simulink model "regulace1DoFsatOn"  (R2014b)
settings: Solver=ode45  StartTime=0.0  StopTime=50  RelTol=1e-3
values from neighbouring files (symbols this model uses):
  p = [0.2728 0.1079 0.3077 0.0546]    [SITOrizeniP.m]    (also in SITOrizeniPD.m; normaHnekonecno.m = [1 (3*alfa(j)-a0)])
  par = [0.2728 0.1079 0.3077 0.0546 0.1370 0.0320 0.1151 0.0357]    [regulace1DoF.m]    (also in SITOrizeniP.m = [-0.0536 0.05 0.13 0.006 -0.0545 0.1 0.16 0.1746 -0.058     ; SITOrizeniPD.m = [-0.0536 0.05 0.13 0.006 -0.0545 0.1 0.16 0.1746 -0.058     ; regulace2DoF.m; regulaceMPM.m)
undefined symbols (not defined in the file or in its folder): magnitude, q
libraries: simulink x4

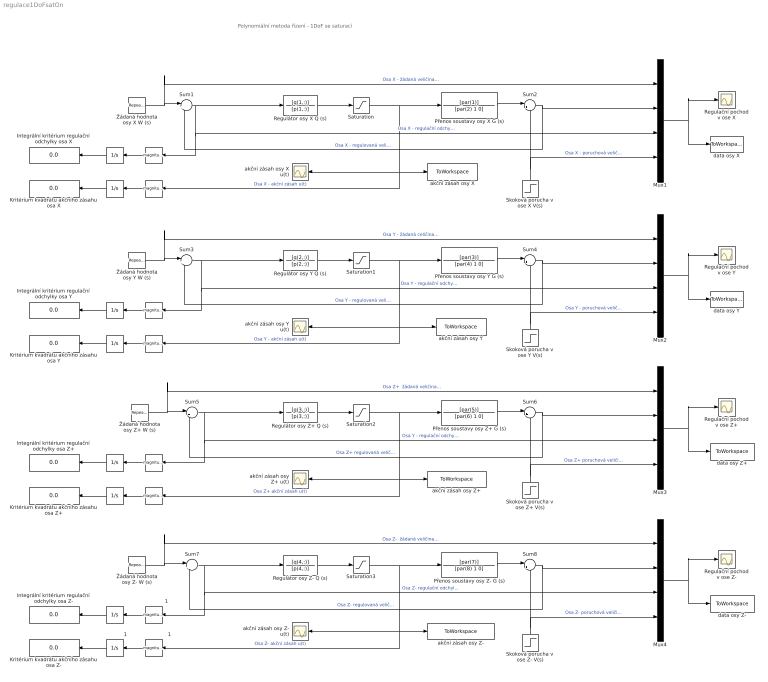
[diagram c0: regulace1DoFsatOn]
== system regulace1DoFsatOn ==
  note: Polynomiální metoda řízení - 1DoF se saturací
  " " : Math  Operator=magnitude^2
  "  " : Integrator
  "    " : Integrator
  "     " : Integrator
  "      " : Math  Operator=magnitude^2
  "        " : Integrator
  "         " : Integrator
  "          " : Math  Operator=magnitude^2
  "             " : Math  Operator=magnitude^2
  "              " : Integrator
  "                 " : Math  Operator=magnitude^2
  "                     " : Math  Operator=magnitude^2
  "                                                  " : Integrator
  "                     1" : Math  Operator=magnitude^2
  "                 1" : Math  Operator=magnitude^2
  "              1" : Integrator
  Integrální kritérium regulační odchylky osa X : Display
  Integrální kritérium regulační odchylky osa Y : Display
  Integrální kritérium regulační odchylky osa Z+ : Display
  Integrální kritérium regulační odchylky osa Z- : Display
  Kritérium kvadrátu akčního zásahu osa X : Display
  Kritérium kvadrátu akčního zásahu osa Y : Display
  Kritérium kvadrátu akčního zásahu osa Z+ : Display
  Kritérium kvadrátu akčního zásahu osa Z- : Display
  Mux{1..4} (4 alike) : Mux
  Přenos soustavy osy X G (s) : TransferFcn  Numerator=[par(1)]  Denominator=[par(2) 1 0]
  Přenos soustavy osy Y G (s) : TransferFcn  Numerator=[par(3)]  Denominator=[par(4) 1 0]
  Přenos soustavy osy Z+ G (s) : TransferFcn  Numerator=[par(5)]  Denominator=[par(6) 1 0]
  Přenos soustavy osy Z- G (s) : TransferFcn  Numerator=[par(7)]  Denominator=[par(8) 1 0]
  Regulační pochod v ose X : Scope
  Regulační pochod v ose Y : Scope
  Regulační pochod v ose Z+ : Scope
  Regulační pochod v ose Z- : Scope
  Regulátor osy X Q (s) : TransferFcn  Numerator=[q(1,:)]  Denominator=[p(1,:)]
  Regulátor osy Y Q (s) : TransferFcn  Numerator=[q(2,:)]  Denominator=[p(2,:)]
  Regulátor osy Z+ Q (s) : TransferFcn  Numerator=[q(3,:)]  Denominator=[p(3,:)]
  Regulátor osy Z- Q (s) : TransferFcn  Numerator=[q(4,:)]  Denominator=[p(4,:)]
  Saturation{,1..3} (4 alike) : Saturate  UpperLimit=1  LowerLimit=-1
  Skoková porucha v ose X V(s) : Step  Time=15  After=0.1  SampleTime=0
  Skoková porucha v ose Y V(s) : Step  Time=15  After=0.1  SampleTime=0
  Skoková porucha v ose Z+ V(s) : Step  Time=15  After=0.1  SampleTime=0
  Skoková porucha v ose Z- V(s) : Step  Time=15  After=0.1  SampleTime=0
  Sum{1,3,5,7} (4 alike) : Sum  Inputs=|+-
  Sum{2,4,6,8} (4 alike) : Sum  Inputs=|++
  akční zásah osy X : ToWorkspace  VariableName=akcniZasahXsat  SaveFormat=Timeseries  SampleTime=-1
  akční zásah osy X u(t) : Scope
  akční zásah osy Y : ToWorkspace  VariableName=akcniZasahYsat  SaveFormat=Timeseries  SampleTime=-1
  akční zásah osy Y u(t) : Scope
  akční zásah osy Z+ : ToWorkspace  VariableName=akcniZasahZplusSat  SaveFormat=Timeseries  SampleTime=-1
  akční zásah osy Z+ u(t) : Scope
  akční zásah osy Z- : ToWorkspace  VariableName=akcniZasahZminusSat  SaveFormat=Timeseries  SampleTime=-1
  akční zásah osy Z- u(t) : Scope
  data osy X : ToWorkspace  VariableName=dataXsat  SaveFormat=Timeseries  SampleTime=-1
  data osy Y : ToWorkspace  VariableName=dataYsat  SaveFormat=Timeseries  SampleTime=-1
  data osy Z+ : ToWorkspace  VariableName=dataZplusSat  SaveFormat=Timeseries  SampleTime=-1
  data osy Z- : ToWorkspace  VariableName=dataZminusSat  SaveFormat=Timeseries  SampleTime=-1
  Žádaná hodnota osy X W (s) : simulink/Sources/Repeating Sequence  rep_seq_t=[0 9.99 10 19.99 20 29.99 30 39.99 40 50]  rep_seq_y=[0 0 0.4 0.4 0.2 0.2 0.6 0.6 0 0]
  Žádaná hodnota osy Y W (s) : simulink/Sources/Repeating Sequence  rep_seq_t=[0 9.99 10 19.99 20 29.99 30 39.99 40 50]  rep_seq_y=[0 0 0.4 0.4 0.2 0.2 0.6 0.6 0 0]
  Žádaná hodnota osy Z+ W (s) : simulink/Sources/Repeating Sequence  rep_seq_t=[0 9.99 10 19.99 20 29.99 30 39.99 40 50]  rep_seq_y=[0 0 0.4 0.4 0.2 0.2 0.6 0.6 0 0]
  Žádaná hodnota osy Z- W (s) : simulink/Sources/Repeating Sequence  rep_seq_t=[0 9.99 10 19.99 20 29.99 30 39.99 40 50]  rep_seq_y=[0 0 0.4 0.4 0.2 0.2 0.6 0.6 0 0]
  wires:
  Žádaná hodnota osy X W (s)/1 -> Sum1/1, Mux1/1  "Osa X - žádaná veličina w(t)"
  Sum1/1 -> Regulátor osy X Q (s)/1, Mux1/3, "      "/1  "Osa X - regulační odchylka e(t)"
  Přenos soustavy osy X G (s)/1 -> Sum2/1
  Sum2/1 -> Sum1/2, Mux1/2  "Osa X - regulovaná veličina y(t)"
  Skoková porucha v ose X V(s)/1 -> Mux1/4, Sum2/2  "Osa X - poruchová veličina v(t)"
  Mux1/1 -> data osy X/1, Regulační pochod v ose X/1
  "      "/1 -> "  "/1
  "  "/1 -> Integrální kritérium regulační odchylky osa X/1
  "     "/1 -> Kritérium kvadrátu akčního zásahu osa X/1
  " "/1 -> "     "/1
  Saturation/1 -> Přenos soustavy osy X G (s)/1, akční zásah osy X/1, " "/1, akční zásah osy X u(t)/1  "Osa X - akční zásah u(t)"
  Regulátor osy X Q (s)/1 -> Saturation/1
  Žádaná hodnota osy Y W (s)/1 -> Sum3/1, Mux2/1  "Osa Y - žádaná celičina w(t)"
  Sum3/1 -> Regulátor osy Y Q (s)/1, Mux2/3, "          "/1  "Osa Y - regulační odchylka e(t)"
  Přenos soustavy osy Y G (s)/1 -> Sum4/1
  Sum4/1 -> Sum3/2, Mux2/2  "Osa Y - regulovaná veličina y(t)"
  Skoková porucha v ose Y V(s)/1 -> Mux2/4, Sum4/2  "Osa Y - poruchová veličina v(t)"
  Mux2/1 -> data osy Y/1, Regulační pochod v ose Y/1
  "          "/1 -> "    "/1
  "    "/1 -> Integrální kritérium regulační odchylky osa Y/1
  "        "/1 -> Kritérium kvadrátu akčního zásahu osa Y/1
  "             "/1 -> "        "/1
  Saturation1/1 -> Přenos soustavy osy Y G (s)/1, akční zásah osy Y/1, "             "/1, akční zásah osy Y u(t)/1  "Osa Y - akční zásah u(t)"
  Regulátor osy Y Q (s)/1 -> Saturation1/1
  Žádaná hodnota osy Z+ W (s)/1 -> Sum5/1, Mux3/1  "Osa Z+  žádaná veličina w(t)"
  Sum5/1 -> Regulátor osy Z+ Q (s)/1, Mux3/3, "                 "/1  "Osa Y - regulační odchylka e(t)"
  Přenos soustavy osy Z+ G (s)/1 -> Sum6/1
  Sum6/1 -> Sum5/2, Mux3/2  "Osa Z+ regulovaná veličina y(t)"
  Skoková porucha v ose Z+ V(s)/1 -> Mux3/4, Sum6/2  "Osa Z+ poruchová veličina v(t)"
  Mux3/1 -> data osy Z+/1, Regulační pochod v ose Z+/1
  "                 "/1 -> "         "/1
  "         "/1 -> Integrální kritérium regulační odchylky osa Z+/1
  "              "/1 -> Kritérium kvadrátu akčního zásahu osa Z+/1
  "                     "/1 -> "              "/1
  Saturation2/1 -> Přenos soustavy osy Z+ G (s)/1, akční zásah osy Z+/1, "                     "/1, akční zásah osy Z+ u(t)/1  "Osa Z+ akční zásah u(t)"
  Regulátor osy Z+ Q (s)/1 -> Saturation2/1
  Žádaná hodnota osy Z- W (s)/1 -> Sum7/1, Mux4/1  "Osa Z-  žádaná veličina w(t)"
  Sum7/1 -> Regulátor osy Z- Q (s)/1, "                 1"/1, Mux4/3  "Osa Z- regulační odchylka e(t)"
  Přenos soustavy osy Z- G (s)/1 -> Sum8/1
  Sum8/1 -> Sum7/2, Mux4/2  "Osa Z- regulovaná veličina y(t)"
  Skoková porucha v ose Z- V(s)/1 -> Mux4/4, Sum8/2  "Osa Z- poruchová veličina v(t)"
  Mux4/1 -> data osy Z-/1, Regulační pochod v ose Z-/1
  "                 1"/1 -> "                                                  "/1
  "                                                  "/1 -> Integrální kritérium regulační odchylky osa Z-/1
  "              1"/1 -> Kritérium kvadrátu akčního zásahu osa Z-/1
  "                     1"/1 -> "              1"/1
  Saturation3/1 -> Přenos soustavy osy Z- G (s)/1, akční zásah osy Z-/1, "                     1"/1, akční zásah osy Z- u(t)/1  "Osa Z- akční zásah u(t)"
  Regulátor osy Z- Q (s)/1 -> Saturation3/1
